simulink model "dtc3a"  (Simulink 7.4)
settings: Solver=ode23  StartTime=0.0  StopTime=2  MaxStep=3e-6  RelTol=1e-3
InitFcn:
  | warning off; wmo=0.0%initial speed
  | fso=1.0 %initial stator flux
undefined symbols (not defined in the file or in its folder): a, wmo

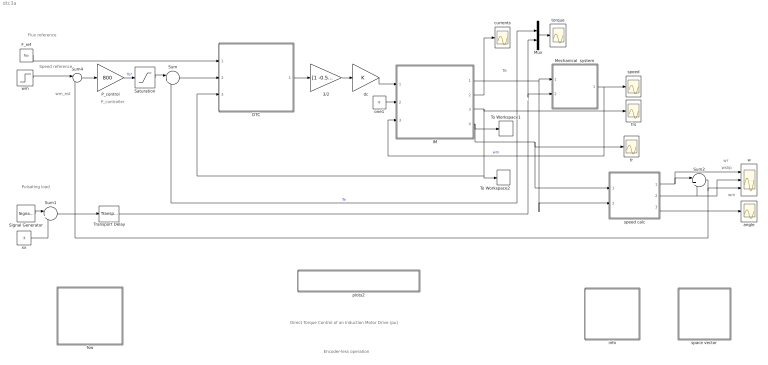
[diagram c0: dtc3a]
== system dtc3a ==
  note: Direct Torque Control of an Induction Motor Drive (pu)
  note: Flux reference
  note: Speed reference
  note: Te
  note: Tl
  note: Pulsating load
  note: P_controller
  note: Encoder-less operation
  note: wm_est
  note: wm
  note: wslip
  note: wr
  3/2 : Gain  Gain=[1 -0.5 -0.5;0 sqrt(3)/2 -sqrt(3)/2]  Multiplication=Matrix(K*u)  ParameterDataType=sfix(16)  ParameterScaling=2^0  OutDataType=sfix(16)  OutScaling=2^0
  DTC : Subsystem
  F_ref : Constant  Value=fso  OutDataType=sfix(16)  OutScaling=2^0
  IM : Subsystem  mask{Rs=0.01, Rr=0.02, Lsl=0.10, Lrl=0.10, Lm=4.5, wo=2*pi*60}
      mask prompts: Rs "Stator resistance [pu]"; Rr "Rotor resistance [pu]"; Lsl "Stator leakage inductance [pu]"; Lrl "Rotor leakage inductance [pu]"; Lm "Magnetizing inductance [pu]"; wo "Base frequency [rad/s]"
  Mechanical  system : Subsystem  mask{H=0.5, Bm=1e-5}
      mask prompts: H "Inertia constant [s]"; Bm "Torque-speed coefficient"
  Mux : Mux  Inputs=2
  P_control : Gain  Gain=800  ParameterDataType=sfix(16)  ParameterScaling=2^0  OutDataType=sfix(16)  OutScaling=2^0
  Saturation : Saturate  UpperLimit=2  LowerLimit=-2
  Signal Generator : SignalGenerator  WaveForm=square  Amplitude=.5  Frequency=4
  Sum : Sum  Inputs=|+-  OutDataType=sfix(16)  OutScaling=2^0
  Sum1 : Sum  Inputs=|++  OutDataType=sfix(16)  OutScaling=2^0
  Sum2 : Sum  Inputs=|+-  OutDataType=sfix(16)  OutScaling=2^0
  Sum4 : Sum  Inputs=|+-  OutDataType=sfix(16)  OutScaling=2^0
  To Workspace1 : ToWorkspace  VariableName=fr  SampleTime=-1  SaveFormat=Array
  To Workspace2 : ToWorkspace  VariableName=fs  SampleTime=-1  SaveFormat=Array
  Transport Delay : TransportDelay
  angle : Scope
  currents : Scope
  dc : Gain  ParameterDataType=sfix(16)  ParameterScaling=2^0  OutDataType=sfix(16)  OutScaling=2^0
  fr : Scope
  frs : Scope
  fsw : Subsystem
  info : Subsystem
  one1 : Constant  Value=0  OutDataType=sfix(16)  OutScaling=2^0
  plots2 : Subsystem
  space vector : Subsystem
  speed : Scope
  speed calc : Subsystem
  torque : Scope
  w : Scope  NumInputPorts=3
  wm : Step  Time=.2  Before=wmo  After=.8  SampleTime=0
  xx : Constant  Value=.5  OutDataType=sfix(16)  OutScaling=2^0
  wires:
  DTC/1(s3) -> 3/2/1
  F_ref/1 -> DTC/1(f_ref)
  3/2/1 -> dc/1
  IM/3(fs) -> To Workspace2/1, DTC/3(fs), frs/1
  one1/1 -> IM/2(wk)
  IM/1(Te) -> Sum/2, Mux/1, Mechanical  system/1(Te), speed calc/2(Te)  "Te"
  Mechanical  system/1(wm) -> speed/1, IM/3(wm)  "wm"
  IM/2(is) -> currents/1
  wm/1 -> Sum4/1
  Sum/1 -> DTC/2(T_er)
  Mux/1 -> torque/1
  Sum4/1 -> P_control/1
  P_control/1 -> Saturation/1  "Te*"
  IM/4(fr) -> To Workspace1/1, fr/1, speed calc/1(fr)
  dc/1 -> IM/1(vs)
  Signal Generator/1 -> Sum1/1
  xx/1 -> Sum1/2
  Sum1/1 -> Transport Delay/1
  Transport Delay/1 -> Mux/2, Mechanical  system/2(Tl)
  Saturation/1 -> Sum/1
  speed calc/1(wr) -> Sum2/1, w/1
  speed calc/2(wslip) -> Sum2/2, w/2
  Sum2/1 -> w/3, Sum4/2
  speed calc/3(an) -> angle/1

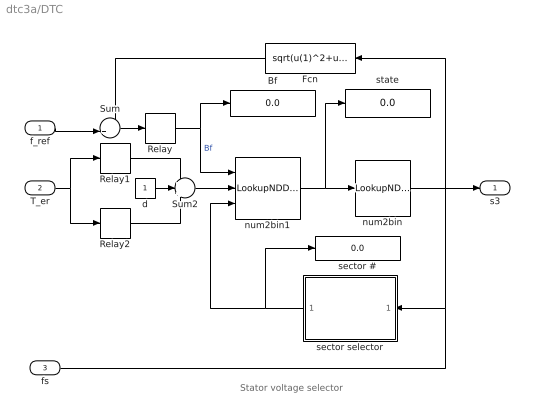
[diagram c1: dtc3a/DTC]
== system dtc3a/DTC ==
  note: Stator voltage selector
  f_ref : Inport  OutDataType=sfix(16)  OutScaling=2^0
  T_er : Inport  Port=2  OutDataType=sfix(16)  OutScaling=2^0
  fs : Inport  Port=3  OutDataType=sfix(16)  OutScaling=2^0
  Bf : Display
  Fcn : Fcn  Expr=sqrt(u(1)^2+u(2)^2)
  Relay : Relay  OnSwitchValue=.01  OffSwitchValue=-.01  OutDataType=sfix(16)  OutScaling=2^0
  Relay1 : Relay  OnSwitchValue=.02  OffSwitchValue=0  OutDataType=sfix(16)  OutScaling=2^0  ZeroCross=off
  Relay2 : Relay  OnSwitchValue=0  OffSwitchValue=-.02  OnOutputValue=0  OffOutputValue=-1  OutDataType=sfix(16)  OutScaling=2^0
  Sum : Sum  Inputs=-+|  OutDataType=sfix(16)  OutScaling=2^0
  Sum2 : Sum  Inputs=+++  OutDataType=sfix(16)  OutScaling=2^0
  d : Constant  OutDataType=sfix(16)  OutScaling=2^0
  num2bin : LookupNDDirect  InputsSelectThisObjectFromTable=Column  Table=[0 0 0;1 0 0;0 1 0;1 1 0;0 0 1;1 0 1;0 1 1;1 1 1]'  ActionForOutOfRangeInput=Error
  num2bin1 : LookupNDDirect  NumberOfTableDimensions=3  Table=a  ActionForOutOfRangeInput=Error
  sector # : Display
  sector selector : Subsystem
  state : Display
  s3 : Outport
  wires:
  num2bin1/1 -> state/1, num2bin/1
  Sum/1 -> Relay/1
  Relay/1 -> Bf/1, num2bin1/1  "Bf"
  Fcn/1 -> Sum/1
  Sum2/1 -> num2bin1/2
  Relay1/1 -> Sum2/1
  Relay2/1 -> Sum2/3
  d/1 -> Sum2/2
  T_er/1 -> Relay2/1, Relay1/1
  f_ref/1 -> Sum/2
  num2bin/1 -> s3/1
  fs/1 -> Fcn/1, sector selector/1(fs)
  sector selector/1(sector) -> num2bin1/3, sector #/1

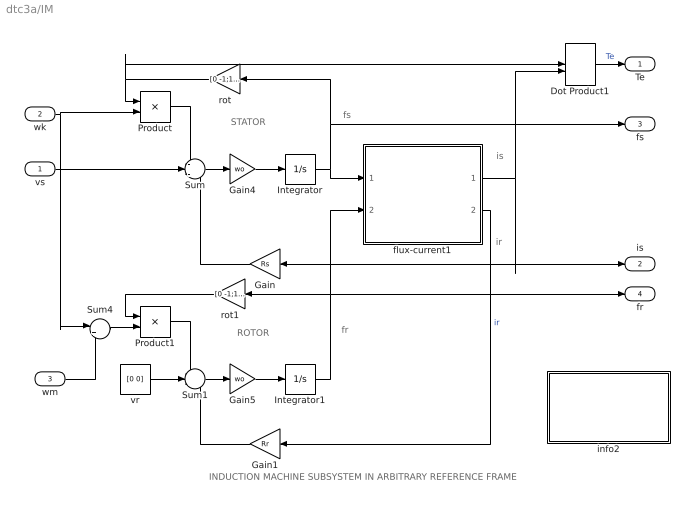
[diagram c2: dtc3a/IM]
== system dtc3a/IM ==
  note: ROTOR
  note: STATOR
  note: fs
  note: fr
  note: is
  note: INDUCTION MACHINE SUBSYSTEM IN ARBITRARY REFERENCE FRAME
  note: ir
  vs : Inport  OutDataType=sfix(16)  OutScaling=2^0
  wk : Inport  Port=2  OutDataType=sfix(16)  OutScaling=2^0
  wm : Inport  Port=3  OutDataType=sfix(16)  OutScaling=2^0
  Dot Product1 : DotProduct  OutDataType=fixdt(1, 16)  OutScaling=2^-10
  Gain : Gain  Gain=Rs  ParameterDataType=sfix(16)  ParameterScaling=2^0  OutDataType=sfix(16)  OutScaling=2^0
  Gain1 : Gain  Gain=Rr  ParameterDataType=sfix(16)  ParameterScaling=2^0  OutDataType=sfix(16)  OutScaling=2^0
  Gain4 : Gain  Gain=wo  ParameterDataType=sfix(16)  ParameterScaling=2^0  OutDataType=sfix(16)  OutScaling=2^0
  Gain5 : Gain  Gain=wo  ParameterDataType=sfix(16)  ParameterScaling=2^0  OutDataType=sfix(16)  OutScaling=2^0
  Integrator : Integrator  InitialCondition=[fso 0]
  Integrator1 : Integrator  InitialCondition=[fso 0]
  Product : Product  OutDataType=sfix(16)  OutScaling=2^0
  Product1 : Product  OutDataType=sfix(16)  OutScaling=2^0
  Sum : Sum  Inputs=-+-  OutDataType=sfix(16)  OutScaling=2^0
  Sum1 : Sum  Inputs=-+-  OutDataType=sfix(16)  OutScaling=2^0
  Sum4 : Sum  Inputs=|+-  OutDataType=sfix(16)  OutScaling=2^0
  flux-current1 : Subsystem
  info2 : Subsystem
  rot : Gain  Gain=[0 -1;1 0]  Multiplication=Matrix(K*u)  ParameterDataType=sfix(16)  ParameterScaling=2^0  OutDataType=sfix(16)  OutScaling=2^0
  rot1 : Gain  Gain=[0 -1;1 0]  Multiplication=Matrix(K*u)  ParameterDataType=sfix(16)  ParameterScaling=2^0  OutDataType=sfix(16)  OutScaling=2^0
  vr : Constant  Value=[0 0]  OutDataType=sfix(16)  OutScaling=2^0
  Te : Outport
  is : Outport  Port=2
  fs : Outport  Port=3
  fr : Outport  Port=4
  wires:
  Gain/1 -> Sum/3
  vr/1 -> Sum1/2
  Gain1/1 -> Sum1/3
  flux-current1/2(ir) -> Gain1/1  "ir"
  Integrator/1 -> flux-current1/1(fs), rot/1, fs/1
  Integrator1/1 -> flux-current1/2(fr), rot1/1, fr/1
  Product1/1 -> Sum1/1
  rot1/1 -> Product1/1
  Product/1 -> Sum/1
  rot/1 -> Product/1, Dot Product1/1
  Sum4/1 -> Product1/2
  Sum/1 -> Gain4/1
  Gain4/1 -> Integrator/1
  Sum1/1 -> Gain5/1
  Gain5/1 -> Integrator1/1
  flux-current1/1(is) -> Gain/1, is/1, Dot Product1/2
  Dot Product1/1 -> Te/1  "Te"
  vs/1 -> Sum/2
  wk/1 -> Product/2, Sum4/1
  wm/1 -> Sum4/2

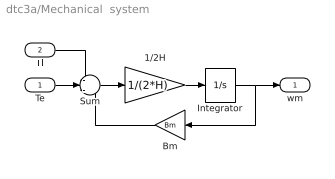
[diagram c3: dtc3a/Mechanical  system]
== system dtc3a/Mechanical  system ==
  Te : Inport  OutDataType=sfix(16)  OutScaling=2^0
  Tl : Inport  Port=2  OutDataType=sfix(16)  OutScaling=2^0
  1/2H : Gain  Gain=1/(2*H)  ParameterDataType=sfix(16)  ParameterScaling=2^0  OutDataType=sfix(16)  OutScaling=2^0
  Bm : Gain  Gain=Bm  ParameterDataType=sfix(16)  ParameterScaling=2^0  OutDataType=sfix(16)  OutScaling=2^0
  Integrator : Integrator  InitialCondition=wmo
  Sum : Sum  Inputs=-+-  OutDataType=sfix(16)  OutScaling=2^0
  wm : Outport
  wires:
  Tl/1 -> Sum/1
  Te/1 -> Sum/2
  Integrator/1 -> wm/1, Bm/1
  Bm/1 -> Sum/3
  Sum/1 -> 1/2H/1
  1/2H/1 -> Integrator/1

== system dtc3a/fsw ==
  note: Script files
  note: This collection of demonstrations is designed to illustrate the use of MATLAB for the simulation of the steady-state characteristics of ac machines under balanced and unbalanced conditions of operation.

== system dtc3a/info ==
  note: Direct torque control of an induction motordrive
  note: The induction motor operates initially at no load at a speed and a stator flux level specified in a callback of the model properties. The mechanical load torque is initially set at Tl = 0 and the electromagnetic torque Te is set to zero by having stator and rotor space vectors colinear (check the IC's of the flux integrators). Before running, double click the Switching Table block.

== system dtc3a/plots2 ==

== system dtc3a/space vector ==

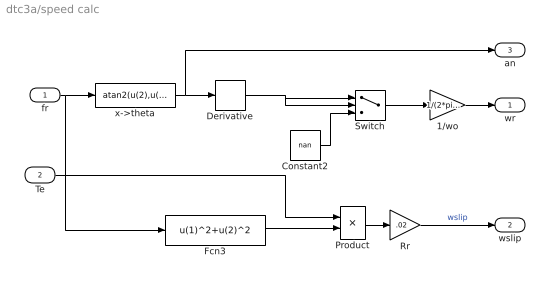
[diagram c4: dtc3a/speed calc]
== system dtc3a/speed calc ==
  fr : Inport  OutDataType=sfix(16)  OutScaling=2^0
  Te : Inport  Port=2  OutDataType=sfix(16)  OutScaling=2^0
  1/wo : Gain  Gain=1/(2*pi*60)  ParameterDataType=sfix(16)  ParameterScaling=2^0  OutDataType=sfix(16)  OutScaling=2^0
  Constant2 : Constant  Value=nan  OutDataType=sfix(16)  OutScaling=2^0
  Derivative : Derivative
  Fcn3 : Fcn  Expr=u(1)^2+u(2)^2
  Product : Product  Inputs=*/  OutDataType=sfix(16)  OutScaling=2^0
  Rr : Gain  Gain=.02  ParameterDataType=sfix(16)  ParameterScaling=2^0  OutDataType=sfix(16)  OutScaling=2^0
  Switch : Switch
  x->theta : Fcn  Expr=atan2(u(2),u(1))
  wr : Outport
  wslip : Outport  Port=2
  an : Outport  Port=3
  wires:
  Switch/1 -> 1/wo/1
  Constant2/1 -> Switch/3
  Derivative/1 -> Switch/1, Switch/2
  fr/1 -> x->theta/1, Fcn3/1
  1/wo/1 -> wr/1
  x->theta/1 -> Derivative/1, an/1
  Fcn3/1 -> Product/2
  Product/1 -> Rr/1
  Te/1 -> Product/1
  Rr/1 -> wslip/1  "wslip"

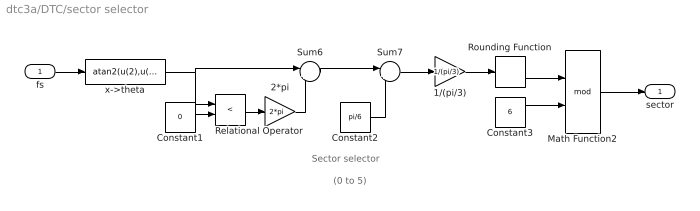
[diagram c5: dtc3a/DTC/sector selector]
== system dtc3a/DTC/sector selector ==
  note: Sector selector
  note: (0 to 5)
  fs : Inport  OutDataType=sfix(16)  OutScaling=2^0
  1/(pi/3) : Gain  Gain=1/(pi/3)  ParameterDataType=sfix(16)  ParameterScaling=2^0  OutDataType=sfix(16)  OutScaling=2^0
  2*pi : Gain  Gain=2*pi  ParameterDataType=sfix(16)  ParameterScaling=2^0  OutDataType=sfix(16)  OutScaling=2^0
  Constant1 : Constant  Value=0  OutDataType=sfix(16)  OutScaling=2^0
  Constant2 : Constant  Value=pi/6  OutDataType=sfix(16)  OutScaling=2^0
  Constant3 : Constant  Value=6  OutDataType=sfix(16)  OutScaling=2^0
  Math Function2 : Math  Operator=mod
  Relational Operator : RelationalOperator  Operator=<
  Rounding Function : Rounding
  Sum6 : Sum  Inputs=|++  OutDataType=sfix(16)  OutScaling=2^0
  Sum7 : Sum  Inputs=|++  OutDataType=sfix(16)  OutScaling=2^0
  x->theta : Fcn  Expr=atan2(u(2),u(1))
  sector : Outport
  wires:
  Constant1/1 -> Relational Operator/2
  Relational Operator/1 -> 2*pi/1
  2*pi/1 -> Sum6/2
  Sum6/1 -> Sum7/1
  Constant2/1 -> Sum7/2
  Sum7/1 -> 1/(pi/3)/1
  1/(pi/3)/1 -> Rounding Function/1
  Rounding Function/1 -> Math Function2/1
  Constant3/1 -> Math Function2/2
  fs/1 -> x->theta/1
  Math Function2/1 -> sector/1
  x->theta/1 -> Relational Operator/1, Sum6/1

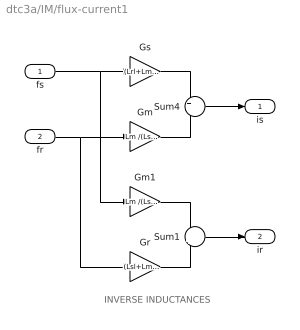
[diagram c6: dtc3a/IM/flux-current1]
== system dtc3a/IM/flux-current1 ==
  note: INVERSE INDUCTANCES
  fs : Inport  OutDataType=sfix(16)  OutScaling=2^0
  fr : Inport  Port=2  OutDataType=sfix(16)  OutScaling=2^0
  Gm : Gain  Gain=Lm /(Lsl*Lrl+Lsl*Lm+Lrl*Lm)  ParameterDataType=sfix(16)  ParameterScaling=2^0  OutDataType=sfix(16)  OutScaling=2^0
  Gm1 : Gain  Gain=Lm /(Lsl*Lrl+Lsl*Lm+Lrl*Lm)  ParameterDataType=sfix(16)  ParameterScaling=2^0  OutDataType=sfix(16)  OutScaling=2^0
  Gr : Gain  Gain=(Lsl+Lm )/(Lsl*Lrl+Lsl*Lm+Lrl*Lm)  ParameterDataType=sfix(16)  ParameterScaling=2^0  OutDataType=sfix(16)  OutScaling=2^0
  Gs : Gain  Gain=(Lrl+Lm) /(Lsl*Lrl+Lsl*Lm+Lrl*Lm)  ParameterDataType=sfix(16)  ParameterScaling=2^0  OutDataType=sfix(16)  OutScaling=2^0
  Sum1 : Sum  Inputs=-+  OutDataType=sfix(16)  OutScaling=2^0
  Sum4 : Sum  Inputs=+-  OutDataType=sfix(16)  OutScaling=2^0
  is : Outport
  ir : Outport  Port=2
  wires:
  fs/1 -> Gs/1, Gm1/1
  Gs/1 -> Sum4/1
  fr/1 -> Gm/1, Gr/1
  Gm/1 -> Sum4/2
  Sum4/1 -> is/1
  Gm1/1 -> Sum1/1
  Gr/1 -> Sum1/2
  Sum1/1 -> ir/1

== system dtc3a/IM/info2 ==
  note: Synchronous machine transients under shortcircuit
  note: This demonstration illustrates the dynamics of a synchronous generator, initially at no load, following a three-phase short circuit at the terminals.
